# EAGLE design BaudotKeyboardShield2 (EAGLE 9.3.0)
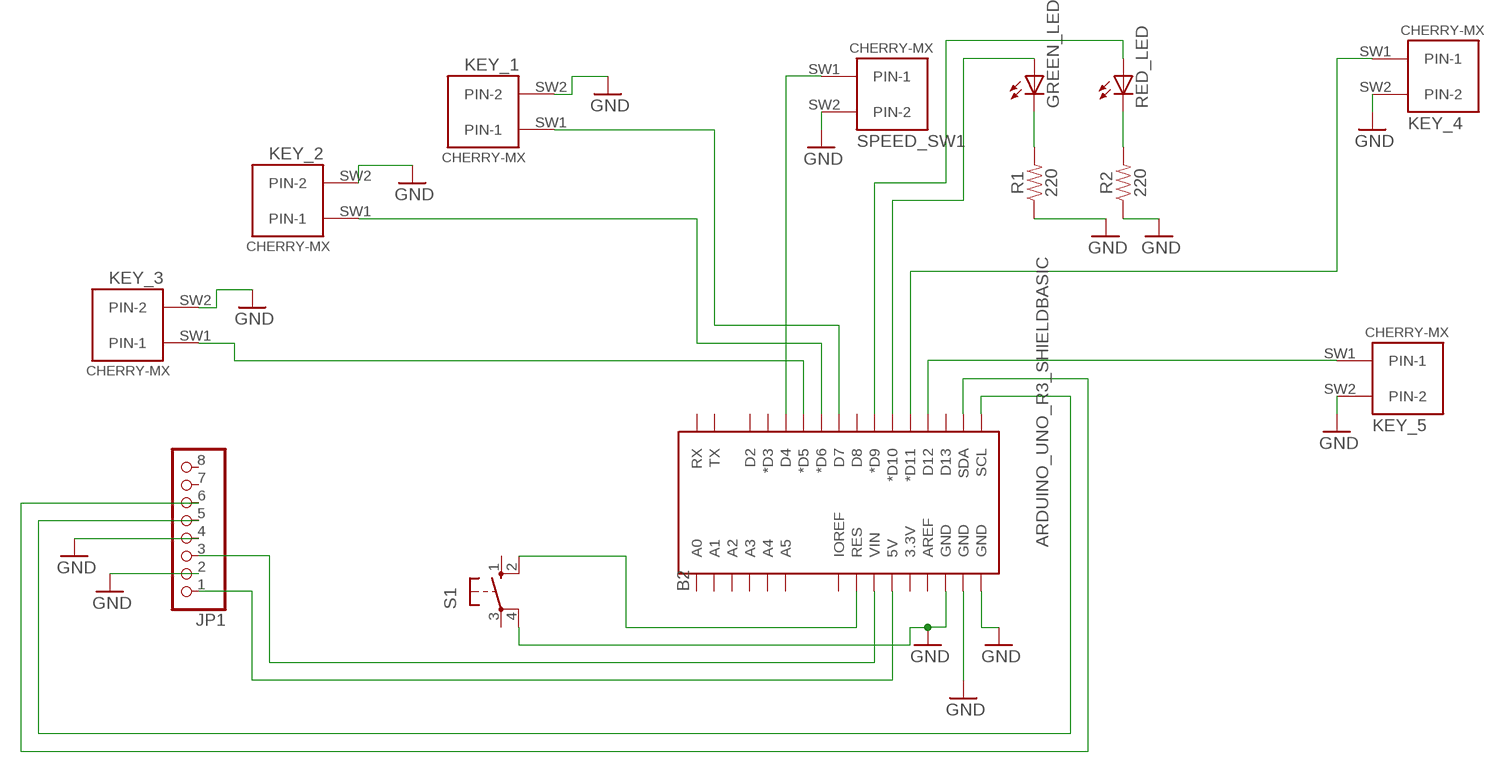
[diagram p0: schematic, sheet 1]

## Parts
B2  ARDUINO_UNO_R3_SHIELDBASIC  [UNO_R3_SHIELD]
GREEN_LED  LED5MM  [LED5MM]
JP1  PINHD-1X8/90  [1X08/90]
KEY_1  CHERRY-MX  [CHERRY-MX]
KEY_2  CHERRY-MX  [CHERRY-MX]
KEY_3  CHERRY-MX  [CHERRY-MX]
KEY_4  CHERRY-MX  [CHERRY-MX]
KEY_5  CHERRY-MX  [CHERRY-MX]
R1  220  100OHM-HORIZ-1/4W-1%  [AXIAL-0.3]
R2  220  100OHM-HORIZ-1/4W-1%  [AXIAL-0.3]
RED_LED  LED5MM  [LED5MM]
S1  10-XX  [B3F-10XX]
SPEED_SW1  CHERRY-MX  [CHERRY-MX]

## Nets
GND: B2.GND@0(GND) B2.GND@1(GND) B2.GND@2(GND) JP1.2 JP1.4 KEY_1.SW2(PIN-2) KEY_2.SW2(PIN-2) KEY_3.SW2(PIN-2) KEY_4.SW2(PIN-2) KEY_5.SW2(PIN-2) R1.P$1 R2.P$1 S1.4(P1) SPEED_SW1.SW2(PIN-2)
N$1: B2.D7 KEY_1.SW1(PIN-1)
N$2: B2.5V JP1.1
N$3: B2.VIN JP1.3
N$4: B2.SCL JP1.5
N$5: B2.SDA JP1.6
N$6: B2.D6(*D6) KEY_2.SW1(PIN-1)
N$7: B2.D5(*D5) KEY_3.SW1(PIN-1)
N$8: B2.D4 SPEED_SW1.SW1(PIN-1)
N$9: GREEN_LED.K(C) R1.P$2
N$10: R2.P$2 RED_LED.K(C)
N$11: B2.D9(*D9) RED_LED.A
N$12: B2.D10(*D10) GREEN_LED.A
N$13: B2.D12 KEY_5.SW1(PIN-1)
N$14: B2.D11(*D11) KEY_4.SW1(PIN-1)
N$15: B2.RES S1.2(S1)
Unconnected: B2.3.3V B2.A0 B2.A1 B2.A2 B2.A3 B2.A4 B2.A5 B2.AREF B2.D2 B2.D3(*D3) B2.D8 B2.D13 B2.IOREF B2.RX B2.TX JP1.7 JP1.8 S1.1(S) S1.3(P)

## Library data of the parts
B2 = SparkFun-Boards:ARDUINO_UNO_R3_SHIELD: Arduino R3 Shield Footprint Shield form compatible with the Arduino Uno R3. SparkFun Products: MG2639 Cellular Shield MIDI Shield R3 Stackable Headers Kit
GREEN_LED RED_LED = adafruit:LED: LED
JP1 = pinhead:PINHD-1X8: PIN HEADER
KEY_1-KEY_5 SPEED_SW1 = cherrymx:CHERRY-MX: Cherry MX series keyswitch
R1 R2 = SparkFun-Resistors:100OHM: 100Ω resistor; PROD_ID: RES-12181; VALUE: 100
S1 = switch-omron:10-XX: OMRON SWITCH; MPN: B3F-1000; OC_FARNELL: 176432; OC_NEWARK: 36M3542

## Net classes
0 default: clearance 0.205 mm

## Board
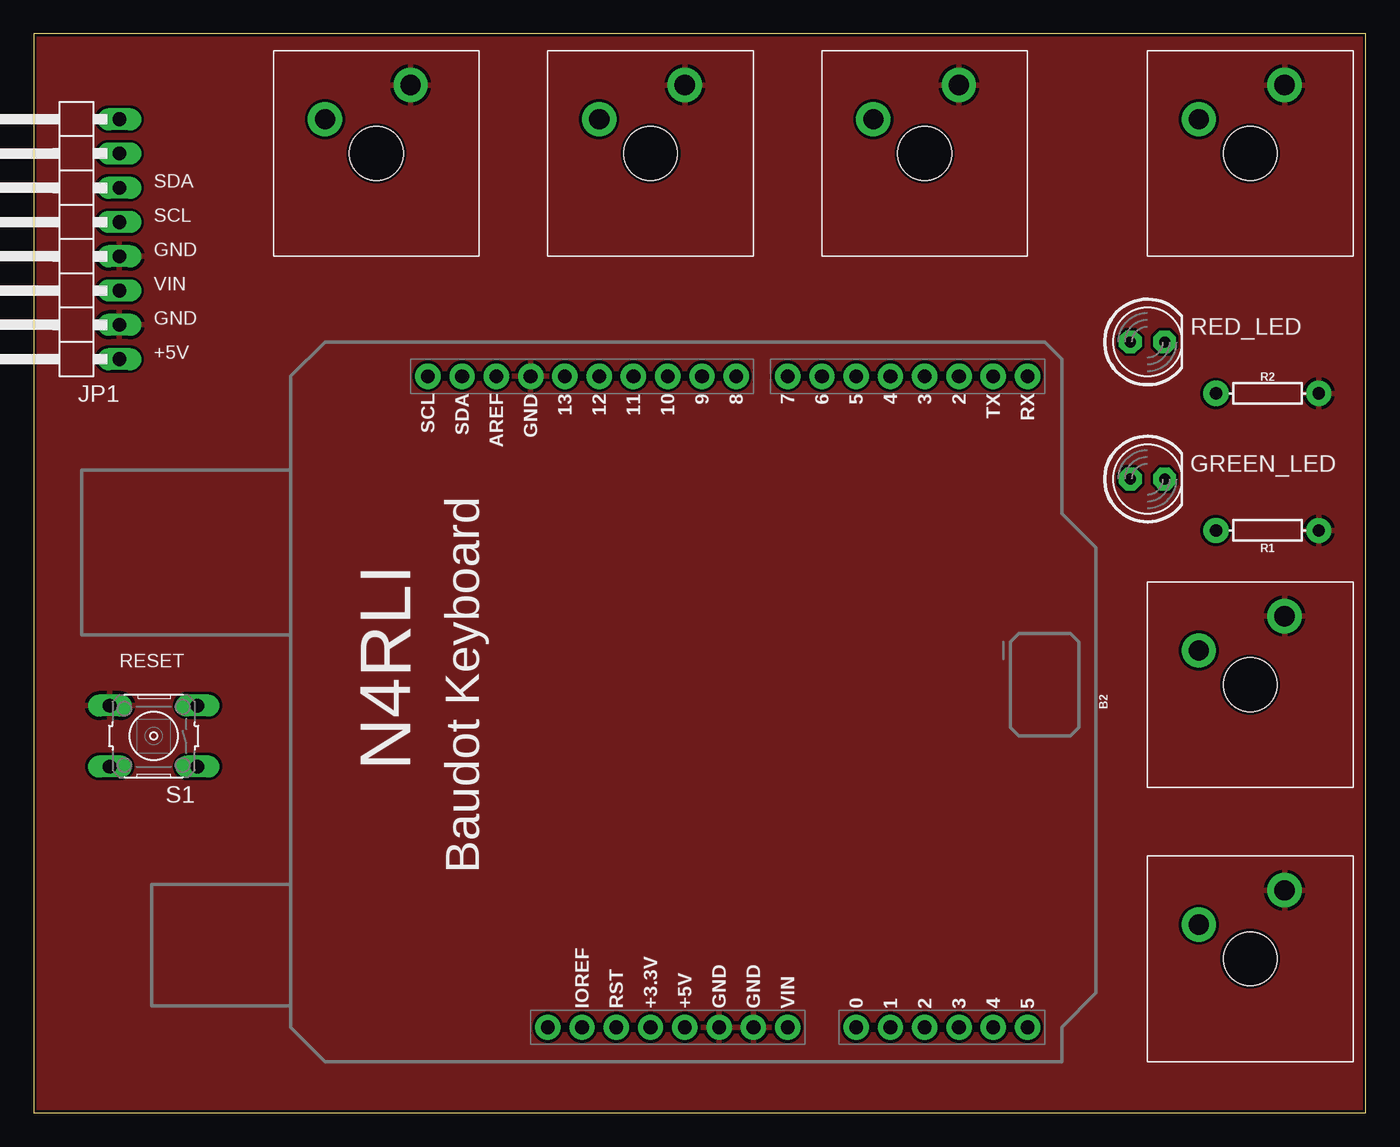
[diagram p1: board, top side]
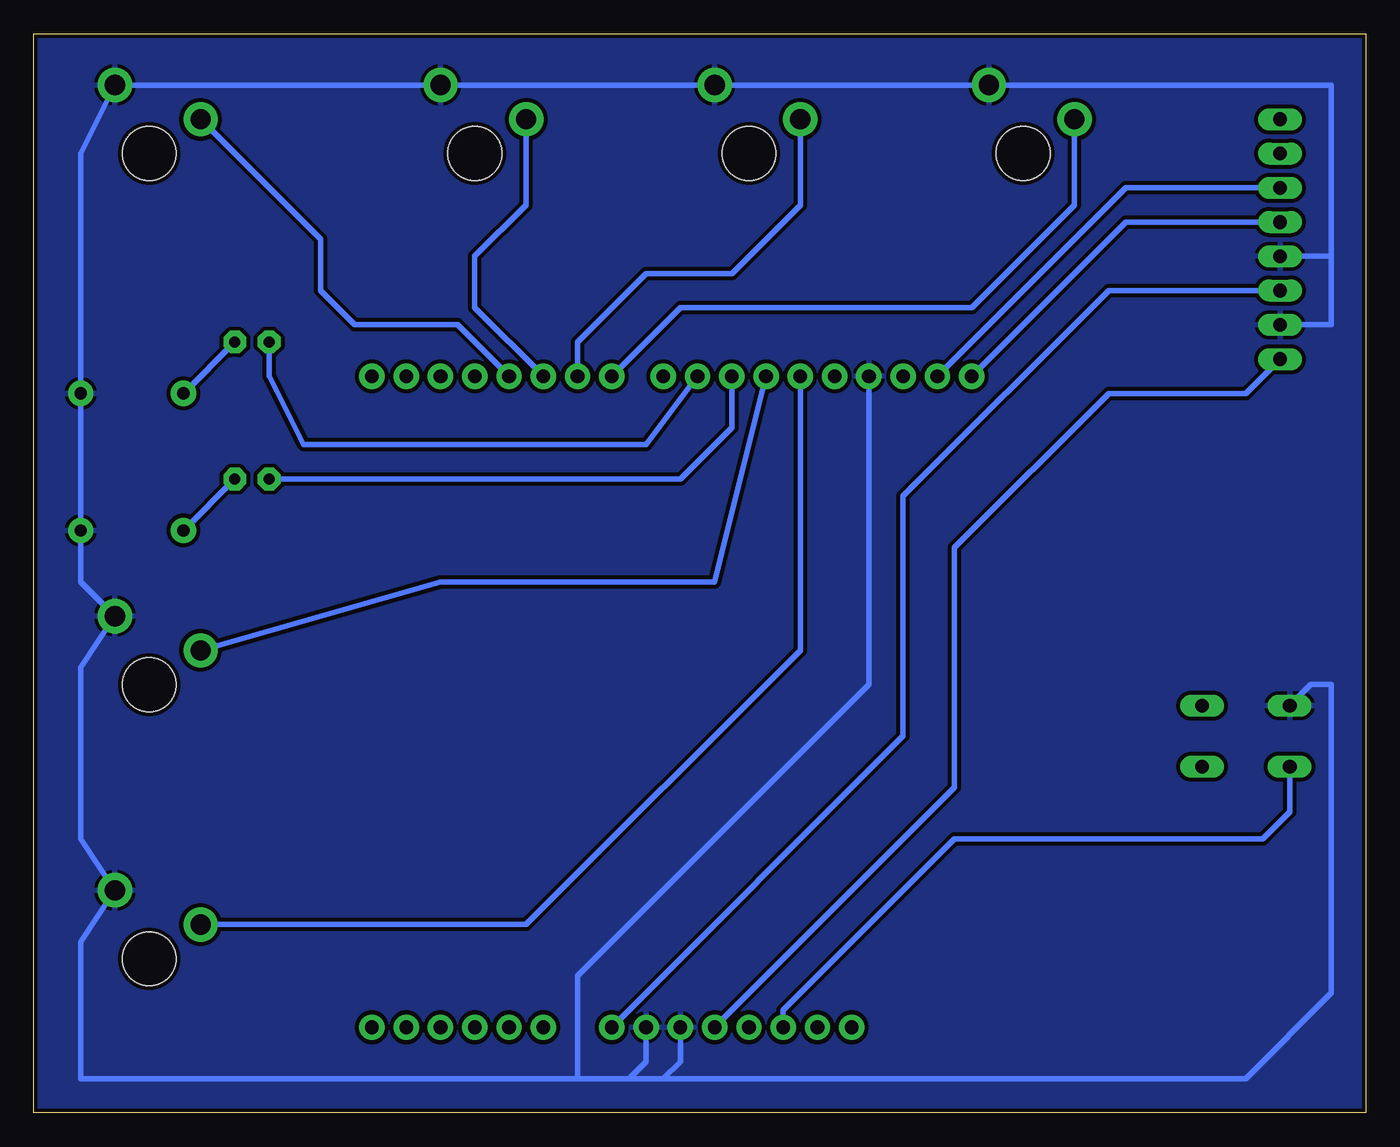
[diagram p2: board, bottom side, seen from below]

Size 98.73 x 80 mm. Coordinates in mm from the lower left corner, seen from the top.
Outline: 0,0 98.73,0 98.73,80 0,80 0,0
Copper layers (1*16): Top 0.035mm / dielectric 1.5mm / Bottom 0.035mm
Design rules "SparkFun": minimum track width 8mil, minimum drill 20mil, track to track 8mil, track to pad 8mil, pad to pad 8mil, via to via 8mil, smd to smd 8mil, copper to edge 8mil, drill to drill 8mil, minimum pad ring 12mil, minimum via ring 10mil, stop-mask expansion 4mil, vias tented up to drill 20mil, thermal gap 10mil

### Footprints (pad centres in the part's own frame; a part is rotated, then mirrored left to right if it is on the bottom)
UNO_R3_SHIELD = drill 1.016 pad 1.88: 3.3V 24.13,-2.54; 5V 24.13,0; A0 24.13,12.7; A1 24.13,15.24; A2 24.13,17.78; A3 24.13,20.32; A4 24.13,22.86; A5 24.13,25.4; AREF -24.13,-13.97; D2 -24.13,20.32; D3 -24.13,17.78; D4 -24.13,15.24; D5 -24.13,12.7; D6 -24.13,10.16; D7 -24.13,7.62; D8 -24.13,3.81; D9 -24.13,1.27; D10 -24.13,-1.27; D11 -24.13,-3.81; D12 -24.13,-6.35; D13 -24.13,-8.89; GND@0 24.13,2.54; GND@1 24.13,5.08; GND@2 -24.13,-11.43; IOREF 24.13,-7.62; NC 24.13,-10.16; RES 24.13,-5.08; RX -24.13,25.4; SCL -24.13,-19.05; SDA -24.13,-16.51; TX -24.13,22.86; VIN 24.13,7.62
LED5MM = drill 0.813 pad 1.676 octagon: A -1.27,0; K 1.27,0
1X08/90 = drill 1.016 long: 1 -8.89,-3.81; 2 -6.35,-3.81; 3 -3.81,-3.81; 4 -1.27,-3.81; 5 1.27,-3.81; 6 3.81,-3.81; 7 6.35,-3.81; 8 8.89,-3.81
CHERRY-MX = drill 1.5 pad 2.54: SW1 -3.81,2.54; SW2 2.54,5.08 | hole 4: 0,0
AXIAL-0.3 = drill 0.9 pad 1.88: P$1 -3.81,0; P$2 3.81,0
B3F-10XX = drill 1.016 long: 1 -3.251,2.261; 2 3.251,2.261; 3 -3.251,-2.261; 4 3.251,-2.261

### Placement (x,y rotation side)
B2  48.26,30.48 270 top
GREEN_LED  82.55,46.99 0 top
JP1  2.54,64.77 90 top
KEY_1  25.4,71.12 0 top
KEY_2  45.72,71.12 0 top
KEY_3  66.04,71.12 0 top
KEY_4  90.17,31.75 0 top
KEY_5  90.17,11.43 0 top
R1  91.44,43.18 180 top
R2  91.44,53.34 180 top
RED_LED  82.55,57.15 0 top
S1  8.89,27.94 180 top
SPEED_SW1  90.17,71.12 0 top

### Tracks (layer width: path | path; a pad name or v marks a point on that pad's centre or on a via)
GND
  Bottom 0.406: 58.42,2.54 95.25,2.54 95.25,12.7 KEY_5.SW2 95.25,20.32 95.25,33.02 KEY_4.SW2 95.25,39.37 R1.P$1 R2.P$1 95.25,71.12 SPEED_SW1.SW2 KEY_3.SW2 KEY_2.SW2 KEY_1.SW2 2.54,76.2 2.54,63.5 | 58.42,2.54 54.61,2.54 | 54.61,2.54 53.34,3.81 B2.GND@1 | B2.GND@0 50.8,3.81 52.07,2.54 | 52.07,2.54 54.61,2.54 | 2.54,63.5 JP1.4 | B2.GND@2 36.83,31.75 58.42,10.16 58.42,2.54 | JP1.2 2.54,58.42 2.54,63.5 | S1.4 4.09,31.75 2.54,31.75 2.54,8.89 8.89,2.54 52.07,2.54
  pour Bottom (isolate 0.305): 1.27,0 0,0 0,80.01 99.06,80.01 99.06,0
  pour Top (isolate 0.305): 1.27,0 0,0 0,80.01 99.06,80.01 99.06,0
  pour Top: 0,80.01 0,-1.27 97.79,-1.27 99.06,0 99.06,80.01
  pour Bottom (isolate 0.305): 0,80.01 0,0 99.06,0 99.06,80.01
N$1
  Bottom 0.406: KEY_1.SW1 21.59,67.31 29.21,59.69 50.8,59.69 B2.D7
N$2
  Bottom 0.406: B2.5V 30.48,24.13 30.48,41.91 19.05,53.34 8.89,53.34 JP1.1
N$3
  Bottom 0.406: B2.VIN 34.29,27.94 34.29,45.72 19.05,60.96 JP1.3
N$4
  Bottom 0.406: B2.SCL 17.78,66.04 JP1.5
N$5
  Bottom 0.406: B2.SDA 17.78,68.58 JP1.6
N$6
  Bottom 0.406: KEY_2.SW1 41.91,67.31 46.99,62.23 53.34,62.23 58.42,57.15 B2.D6
N$7
  Bottom 0.406: KEY_3.SW1 62.23,67.31 66.04,63.5 66.04,59.69 B2.D5
N$8
  Bottom 0.406: SPEED_SW1.SW1 77.47,64.77 77.47,60.96 74.93,58.42 67.31,58.42 B2.D4
N$9
  Bottom 0.406: R1.P$2 GREEN_LED.K
N$10
  Bottom 0.406: RED_LED.K R2.P$2
N$11
  Bottom 0.406: RED_LED.A 81.28,54.61 78.74,49.53 53.34,49.53 B2.D9
N$12
  Bottom 0.406: GREEN_LED.A 50.8,46.99 46.99,50.8 B2.D10
N$13
  Bottom 0.406: KEY_5.SW1 62.23,13.97 41.91,34.29 B2.D12
N$14
  Bottom 0.406: KEY_4.SW1 68.58,39.37 48.26,39.37 B2.D11
N$15
  Bottom 0.406: S1.2 5.64,22.3 7.62,20.32 30.48,20.32 43.18,7.62 B2.RES

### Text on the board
tPlace: SDA | SCL | GND | VIN | GND | +5V | RESET
tNames: N4RLI | Baudot Keyboard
